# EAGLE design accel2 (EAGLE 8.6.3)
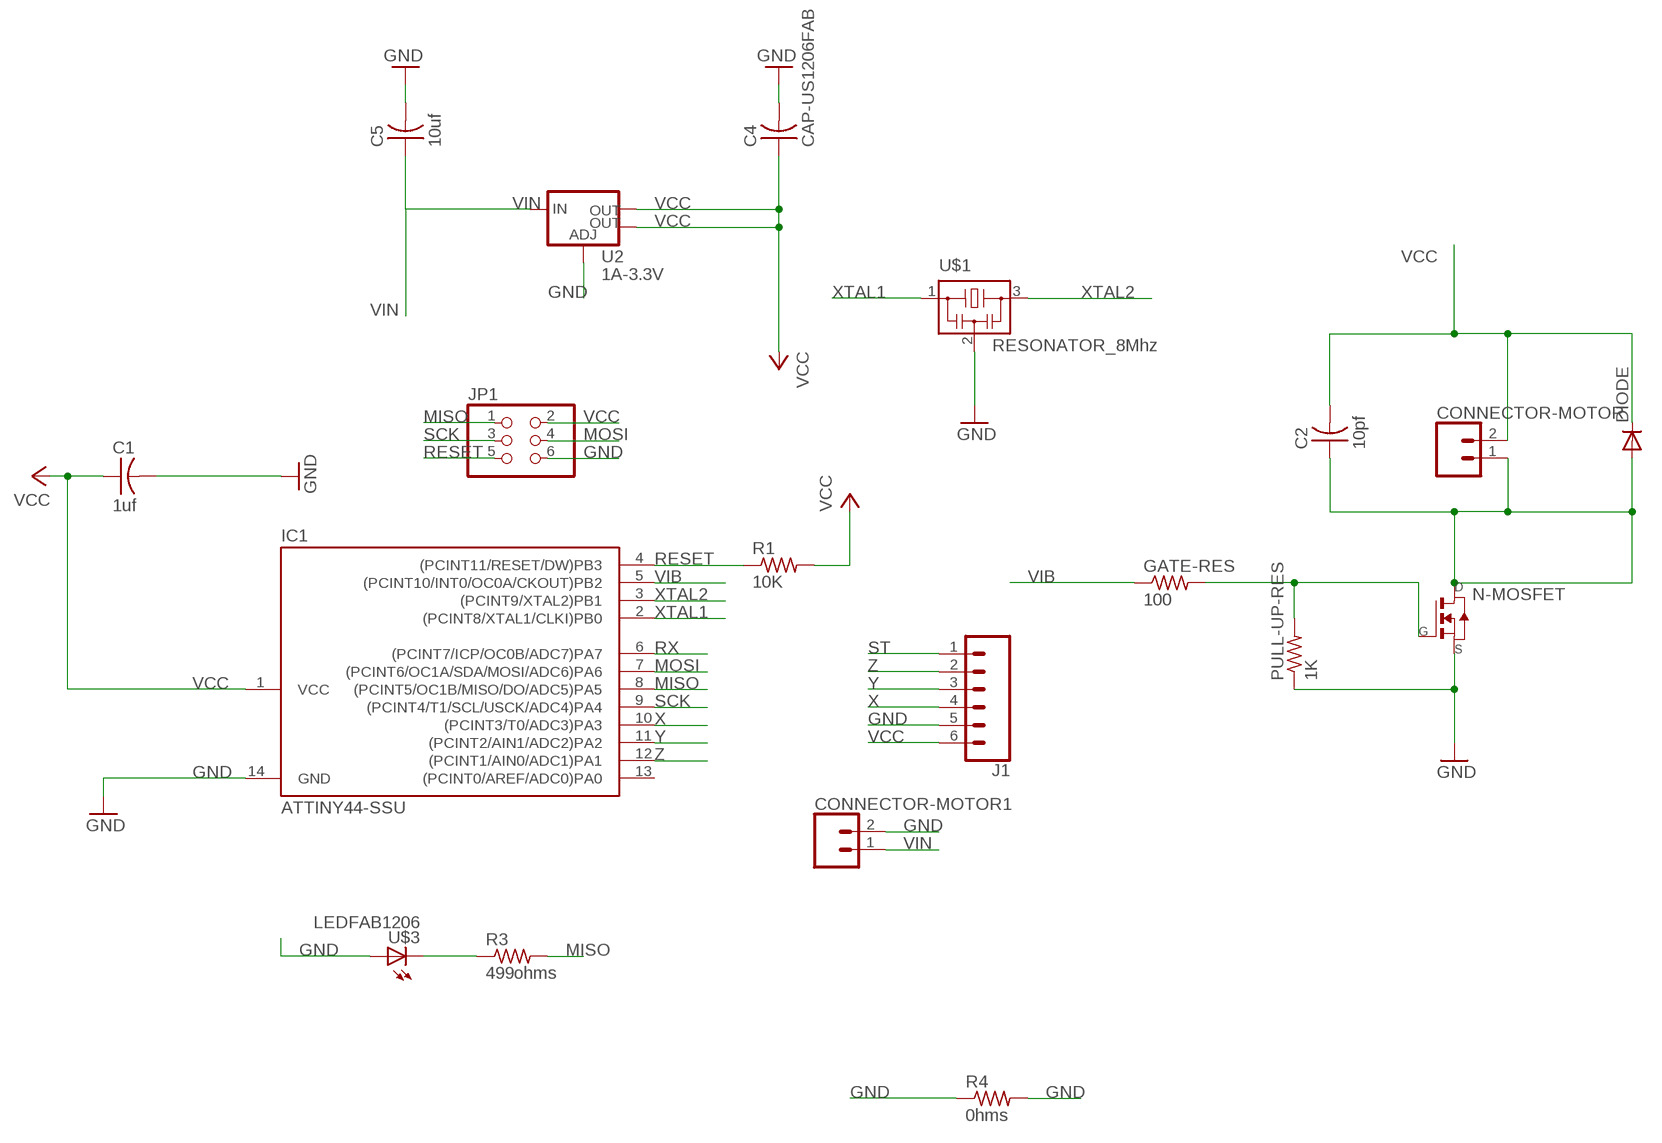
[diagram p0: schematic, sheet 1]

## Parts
C1  1uf  CAP-US1206FAB  [C1206FAB]
C2  10pf  CAP-US1206FAB  [C1206FAB]
C4  CAP-US1206FAB  [C1206FAB]
C5  10uf  CAP-US1206FAB  [C1206FAB]
CONNECTOR-MOTOR  CONN_02PTH3  [1X02_LONGPADS]
CONNECTOR-MOTOR1  CONN_02JST-PTH-2  [JST-2-PTH]
DIODE  DIODESOD123  [SOD123]
GATE-RES  100  RES-US1206FAB  [R1206FAB]
IC1  ATTINY44-SSU  [SOIC14]
J1  CONN_06LONGPADS  [1X06_LONGPADS]
JP1  PINHD-2X3-SMD  [2X03SMD]
N-MOSFET  NMOSFETSOT23  [SOT-23]
PULL-UP-RES  1K  RES-US1206FAB  [R1206FAB]
R1  10K  RES-US1206FAB  [R1206FAB]
R3  499ohms  RES-US1206FAB  [R1206FAB]
R4  0hms  RES-US1206FAB  [R1206FAB]
U2  1A-3.3V  V_REG_LM1117SOT223  [SOT223]
U$1  RESONATOR_8Mhz  RESONATOR  [EFOBM]
U$3  LEDFAB1206  [LED1206FAB]

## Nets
GND: C1.2 C4.2 C5.2 CONNECTOR-MOTOR1.2 IC1.14(GND) J1.5 JP1.6 N-MOSFET.2(S) PULL-UP-RES.1 R4.1 R4.2 U2.1(ADJ) U$1.2 U$3.1(A)
MISO: IC1.8((PCINT5/OC1B/MISO/DO/ADC5)PA5) JP1.1 R3.2
MOSI: IC1.7((PCINT6/OC1A/SDA/MOSI/ADC6)PA6) JP1.4
N$1: C2.1 CONNECTOR-MOTOR.1 DIODE.ANODE(A) N-MOSFET.1(D)
N$2: GATE-RES.2 N-MOSFET.3(G) PULL-UP-RES.2
N$3: R3.1 U$3.2(C)
RESET: IC1.4((PCINT11/RESET/DW)PB3) JP1.5 R1.1
RX: IC1.6((PCINT7/ICP/OC0B/ADC7)PA7)
SCK: IC1.9((PCINT4/T1/SCL/USCK/ADC4)PA4) JP1.3
ST: J1.1
VCC: C1.1 C2.2 C4.1 CONNECTOR-MOTOR.2 DIODE.CATHODE(C) IC1.1(VCC) J1.6 JP1.2 R1.2 U2.2(OUT) U2.4(OUT)
VIB: GATE-RES.1 IC1.5((PCINT10/INT0/OC0A/CKOUT)PB2)
VIN: C5.1 CONNECTOR-MOTOR1.1 U2.3(IN)
X: IC1.10((PCINT3/T0/ADC3)PA3) J1.4
XTAL1: IC1.2((PCINT8/XTAL1/CLKI)PB0) U$1.1
XTAL2: IC1.3((PCINT9/XTAL2)PB1) U$1.3
Y: IC1.11((PCINT2/AIN1/ADC2)PA2) J1.3
Z: IC1.12((PCINT1/AIN0/ADC1)PA1) J1.2
Unconnected: IC1.13((PCINT0/AREF/ADC0)PA0)

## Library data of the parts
C1 C2 C4 C5 = private:CAP-US
CONNECTOR-MOTOR = private:CONN_02: Multi connection point. Often used as Generic Header-pin footprint for 0.1 inch spaced/style header connections
CONNECTOR-MOTOR1 = SparkFun-Connectors:CONN_02: Multi connection point. Often used as Generic Header-pin footprint for 0.1 inch spaced/style header connections; PROD_ID: CONN-09863; SKU: PRT-09914
DIODE = private:DIODE: DIODE
GATE-RES PULL-UP-RES R1 R3 R4 = private:RES-US: Resistor (US Symbol)
IC1 = private:ATTINY44
J1 = SparkFun-Connectors:CONN_06: Multi connection point. Often used as Generic Header-pin footprint for 0.1 inch spaced/style header connections On any of the 0.1 inch spaced packages, you can populate with these: Break Away Headers - Straight (PRT-00116) Break Away Male Headers - Right Angle (PRT-00553) Female Headers (PRT-00115)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
JP1 = private:PINHD-2X3-SMD: PIN HEADER
N-MOSFET = private:NMOSFET: MOS FET
U2 = fab:V_REG_LM1117: Voltage Regulator LM1117 Standard adjustable voltage regulator but in SMD form. Spark Fun Electronics SKU : COM-00595; PROD_ID: VREG-08170
U$1 = private:RESONATOR
U$3 = fab:LED: LED

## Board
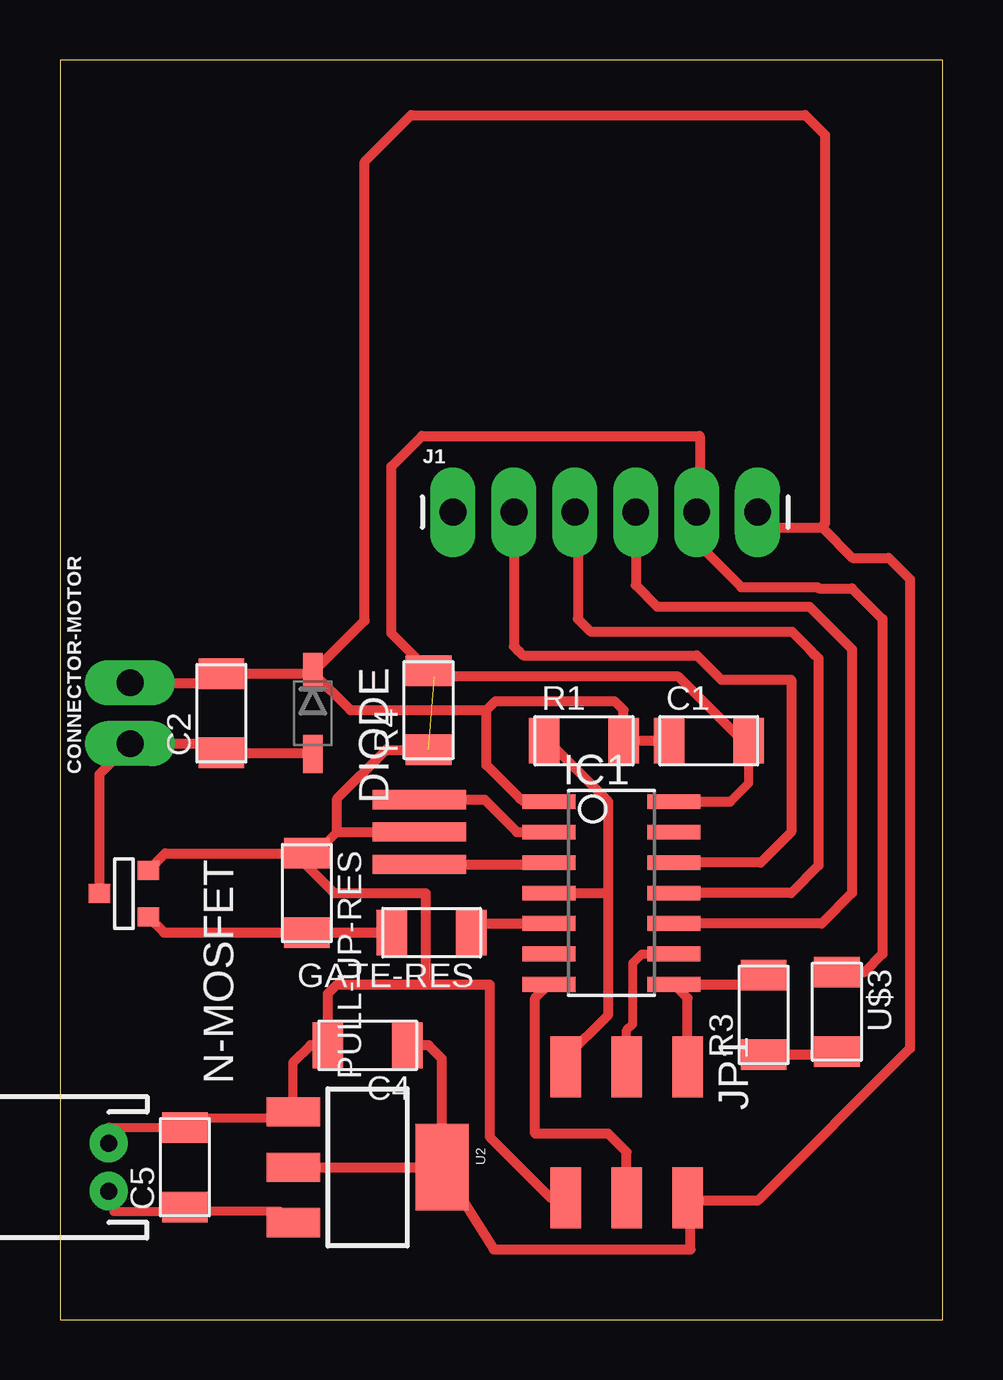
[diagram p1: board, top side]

Size 36.81 x 52.5 mm. Coordinates in mm from the lower left corner, seen from the top.
Outline: 0,0 36.81,0 36.81,52.5 0,52.5 0,0
Copper layers (1*16): Top 0.035mm / dielectric 1.5mm / Bottom 0.035mm
Design rules "default *": minimum track width 15mil, minimum drill 0.79mm, track to track 0.405mm, track to pad 0.405mm, pad to pad 0.405mm, via to via 0.405mm, smd to smd 6mil, copper to edge 40mil, drill to drill 6mil, minimum pad ring 10mil, minimum via ring 8mil, stop-mask expansion 4mil, vias tented up to drill 0mil, thermal gap 10mil

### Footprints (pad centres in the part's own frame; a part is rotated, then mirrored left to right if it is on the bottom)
C1206FAB = smd 1.27 x 1.905: 1 -1.651,0; 2 1.651,0
1X02_LONGPADS = drill 1.118 pad 1.88 long: 1 0,0; 2 2.54,0
JST-2-PTH = drill 0.7 pad 1.6: 1 -1,0; 2 1,0
SOD123 = smd 1.6 x 0.8: ANODE 1.7,0; CATHODE -1.7,0
R1206FAB = smd 1.27 x 1.905: 1 -1.651,0; 2 1.651,0
SOIC14 = smd 0.61 x 2.21: 1 -3.81,-2.603; 2 -2.54,-2.603; 3 -1.27,-2.603; 4 0,-2.603; 5 1.27,-2.603; 6 2.54,-2.603; 7 3.81,-2.603; 8 3.81,2.603; 9 2.54,2.603; 10 1.27,2.603; 11 0,2.603; 12 -1.27,2.603; 13 -2.54,2.603; 14 -3.81,2.603
1X06_LONGPADS = drill 1.118 pad 1.88 long: 1 0,0; 2 2.54,0; 3 5.08,0; 4 7.62,0; 5 10.16,0; 6 12.7,0
2X03SMD = smd 2.54 x 1.27: 1 -2.54,2.54; 2 2.92,2.54; 3 -2.54,0; 4 2.92,0; 5 -2.54,-2.54; 6 2.92,-2.54
SOT-23 = smd 0.787 x 0.889: 1 0.025,-1.016; 2 -0.94,1.016; 3 0.991,1.016
SOT223 = smd 1.219 x 2.235: 1 -2.311,-3.099; 2 0,-3.099; 3 2.311,-3.099 | smd 3.6 x 2.2: 4 0,3.099
EFOBM = smd 0.8 x 3.9: 1 -1.35,0; 2 0,0; 3 1.35,0
LED1206FAB = smd 1.27 x 1.905: 1 -1.651,0; 2 1.651,0

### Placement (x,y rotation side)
C1  27.05,24.13 0 top
C2  6.73,25.27 90 top
C4  12.83,11.43 180 top
C5  5.21,6.35 90 top
CONNECTOR-MOTOR  2.92,24 90 top
CONNECTOR-MOTOR1  2.03,6.35 90 top
DIODE  10.54,25.27 270 top
GATE-RES  15.49,16.13 180 top
IC1  22.99,17.78 270 top
J1  16.38,33.66 0 top
JP1  23.62,8 270 top
N-MOSFET  2.67,17.78 270 top
PULL-UP-RES  10.29,17.78 270 top
R1  21.84,24.13 0 top
R3  29.34,12.7 90 top
R4  15.37,25.4 90 top
U2  12.83,6.35 270 top
U$1  14.99,20.32 270 top
U$3  32.38,12.83 270 top

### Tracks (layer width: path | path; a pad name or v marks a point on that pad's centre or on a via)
GND  (1 unrouted)
  Top 0.381: 11.15,11.05 C4.2 | 9.97,8.8 U2.1 | 4.9,7.63 C5.2 5.29,8.02 | 5.29,8.02 5.68,8.41 9.58,8.41 U2.1 | PULL-UP-RES.1 10.67,19.43 11.56,20.32 | U2.1 9.73,10.72 | CONNECTOR-MOTOR1.2 2.07,8.02 5.29,8.02 | 28.83,24.64 C1.2 28.7,22.35 27.94,21.59
  Top 0.406: C5.2 4.83,7.62 | 15.24,13.97 11.56,13.97 11.18,13.59 C4.2 10.44,11.43 9.73,10.72 | 15.24,13.97 17.91,13.97 17.91,7.62 20.45,5.08 JP1.6 | IC1.14 27.94,21.59 | 15.24,13.97 15.24,17.78 11.43,17.78 10.29,18.92 PULL-UP-RES.1 4.39,19.43 N-MOSFET.2 | R4.1 13.59,23.75 11.56,21.72 11.56,20.32 U$1.2 | U$3.1 33.53,14.48 34.29,15.24 34.29,29.21 33.02,30.48 31.63,30.48 31.58,30.53 28.4,30.53 26.54,32.38 J1.5 26.67,33.53 26.67,36.83 15.09,36.83 13.82,35.56 13.82,28.6 R4.2 15.62,26.8 25.78,26.8 26.92,25.65 27.18,25.4 28.45,24.13 C1.2
MISO
  Top 0.406: JP1.1 26.16,13.4 IC1.8 28.96,13.97 R3.2
MOSI
  Top 0.381: 20.13,14.03 IC1.7
  Top 0.406: JP1.4 23.62,6.99 22.86,7.75 19.81,7.75 19.81,13.4 IC1.7
N$1
  Top 0.406: DIODE.ANODE 10.49,23.62 C2.1 6.35,24 CONNECTOR-MOTOR.1 1.65,22.73 N-MOSFET.1
N$2
  Top 0.406: N-MOSFET.3 4.34,16.13 PULL-UP-RES.2 GATE-RES.2
N$3
  Top 0.406: R3.1 32.26,11.05 U$3.2
RESET
  Top 0.381: 20.32,24.38 R1.1
  Top 0.406: JP1.5 21.08,10.92 22.86,12.7 22.86,17.78 | 22.86,17.78 22.86,21.59 20.32,24.13 R1.1 | IC1.4 22.86,17.78
SCK
  Top 0.381: JP1.3 23.62,12.06 23.88,12.32 23.88,14.86 24.26,15.24 IC1.9
VCC
  Top 0.381: 18.67,22.23 19.18,21.72 19.3,21.59 IC1.1
  Top 0.406: DIODE.CATHODE 10.49,26.92 C2.2 6.35,26.54 CONNECTOR-MOTOR.2 | U2.2 U2.4 | U2.4 15.93,10.87 15.37,11.43 C4.1 | C1.1 R1.2 23.5,25.4 23.11,25.78 18.16,25.78 17.78,25.4 | 31.75,33.04 31.75,33.02 29.72,33.02 J1.6 29.21,33.53 | 31.75,33.04 31.9,33.19 31.9,49.37 31.07,50.2 14.64,50.2 12.7,48.26 12.7,29.13 DIODE.CATHODE | U2.4 18.09,2.92 26.29,2.92 26.29,4.95 | 26.29,4.95 JP1.2 | DIODE.CATHODE 12.11,25.4 17.78,25.4 | 31.75,33.04 33.04,31.75 34.54,31.75 35.43,30.86 35.43,11.3 29.08,4.95 26.29,4.95 | 19.18,21.72 17.78,23.11 17.78,25.4
VIB
  Top 0.406: GATE-RES.1 17.53,16.51 IC1.5
VIN
  Top 0.381: 5.29,4.51 9.19,4.51 9.58,4.12 U2.3 | 5.29,4.51 C5.1 4.9,4.9 | CONNECTOR-MOTOR1.1 2.24,4.51 5.29,4.51
X
  Top 0.406: J1.4 24,30.61 24.89,29.72 31.24,29.72 33.02,27.94 33.02,17.78 31.75,16.51 IC1.10
XTAL1
  Top 0.406: U$1.1 17.7,21.67 19.05,20.32 IC1.2
XTAL2
  Top 0.381: 20.13,19.11 IC1.3
  Top 0.406: U$1.3 20.3,18.97 IC1.3
Y
  Top 0.406: J1.3 21.59,33.53 21.59,29.21 22.14,28.66 30.52,28.66 31.24,27.94 31.5,27.69 31.62,27.56 31.62,18.92 30.48,17.78 IC1.11
Z
  Top 0.406: J1.2 18.92,28.07 19.14,27.85 19.3,27.69 26.54,27.69 27.56,26.67 30.48,26.67 30.48,20.32 29.21,19.05 IC1.12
